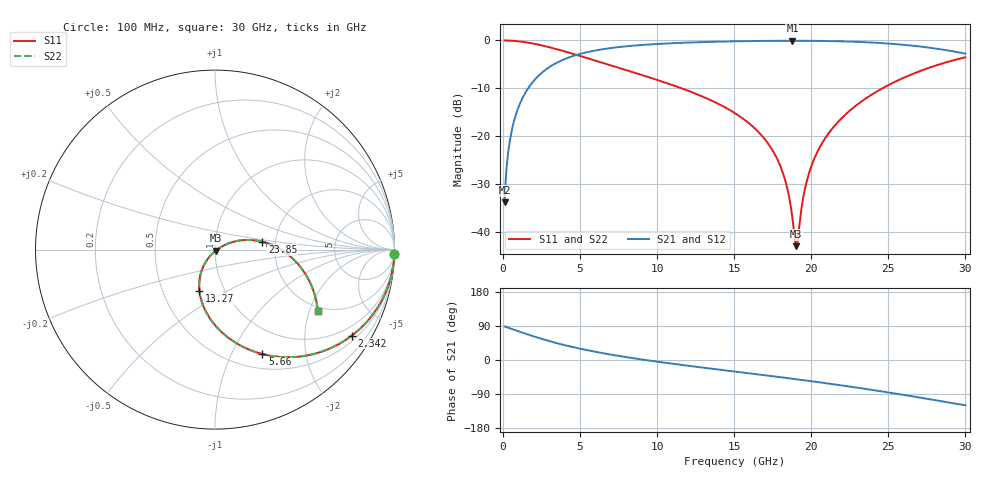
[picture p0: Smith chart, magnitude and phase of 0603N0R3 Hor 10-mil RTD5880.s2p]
# GHz S MA R 50
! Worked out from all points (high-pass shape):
!   3201 points, 100 MHz to 30 GHz, reference 50 ohm
!   highest |S21| = -0.06 dB at 18.78 GHz (marker M1); lowest = -33.8 dB at 100 MHz (marker M2)
!   |S21| within 3 dB of the highest: 4.727 GHz to end of sweep
!   lowest |S11| = -43.0 dB at 19.03 GHz (marker M3), VSWR 1.01, Z = 50.5 - j0.554 ohm
!   |S11| at or under -10 dB: 11.58 GHz to 24.61 GHz (13.03 GHz wide, 72 % of centre)
!   |S22| runs from -43.0 to 0.0 dB; largest |S21 - S12| = 0
!   S11 on the Smith chart (normalised r, x): 100 MHz: 1, -79; 2.342 GHz: 0.66, -3.35; 5.66 GHz: 0.67, -1.32; 13.27 GHz: 0.76, -0.37; 23.85 GHz: 1.71, +0.16; 30 GHz: 1.85, -2.29
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0.1  0.9998 -1.4  0.02046 88.6  0.02046 88.6  0.9998 -1.4
0.4083438  0.9965 -5.9  0.0833 84.1  0.0833 84.1  0.9965 -5.9
0.7914375  0.9871 -11.4  0.16 78.6  0.16 78.6  0.9871 -11.4
1.436156  0.9592 -20.3  0.2825 69.6  0.2825 69.6  0.9592 -20.3
2.3425  0.9005 -32.1  0.434 57.8  0.434 57.8  0.9005 -32.1
3.594562  0.8013 -46.5  0.5971 43.4  0.5971 43.4  0.8013 -46.5
5.089563  0.6817 -60.8  0.7298 29.1  0.7298 29.1  0.6817 -60.8
5.659531  0.6394 -65.6  0.7669 24.3  0.7669 24.3  0.6394 -65.6
10.06978  0.3837 -94.3  0.9199 -4.8  0.9199 -4.8  0.3837 -94.3
13.26534  0.2463 -110.6  0.9645 -21.6  0.9645 -21.6  0.2463 -110.6
15.05  0.1739 -118.8  0.9794 -30.5  0.9794 -30.5  0.1739 -118.8
16.56369  0.1111 -125.1  0.9878 -38.1  0.9878 -38.1  0.1111 -125.1
17.62888  0.06494 -127.9  0.9913 -43.5  0.9913 -43.5  0.06494 -127.9
18.32966  0.03358 -125.5  0.9925 -47.1  0.9925 -47.1  0.03358 -125.5
18.77816  0.01385 -109.2  0.9927 -49.4  0.9927 -49.4  0.01385 -109.2
19.03044  0.007118 -50.5  0.9926 -50.8  0.9926 -50.8  0.007118 -50.5
19.56303  0.027 20.4  0.992 -53.6  0.992 -53.6  0.027 20.4
20.03956  0.05045 25.0  0.9908 -56.2  0.9908 -56.2  0.05045 25.0
21.4785  0.1267 21.9  0.983 -64.2  0.983 -64.2  0.1267 21.9
23.85181  0.2675 9.4  0.9529 -78.3  0.9529 -78.3  0.2675 9.4
25.01978  0.3428 2.4  0.9278 -85.7  0.9278 -85.7  0.3428 2.4
30  0.6676 -30.9  0.7286 -119.5  0.7286 -119.5  0.6676 -30.9
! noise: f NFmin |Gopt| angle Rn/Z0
0.1  0.0007312  0.9801  1.231  0.008369
3.417  0.003821  0.8047  11.33  0.004025
6.743  0.006434  0.7724  19.75  0.005602
10.06  0.008956  0.7584  28.27  0.007066
13.39  0.01162  0.7544  36.75  0.008625
16.7  0.01459  0.7577  45.05  0.01044
20.03  0.01812  0.7673  53.2  0.01272
23.35  0.02247  0.7821  61.16  0.01577
26.67  0.02817  0.802  68.99  0.02016
30  0.03605  0.8263  76.69  0.027
